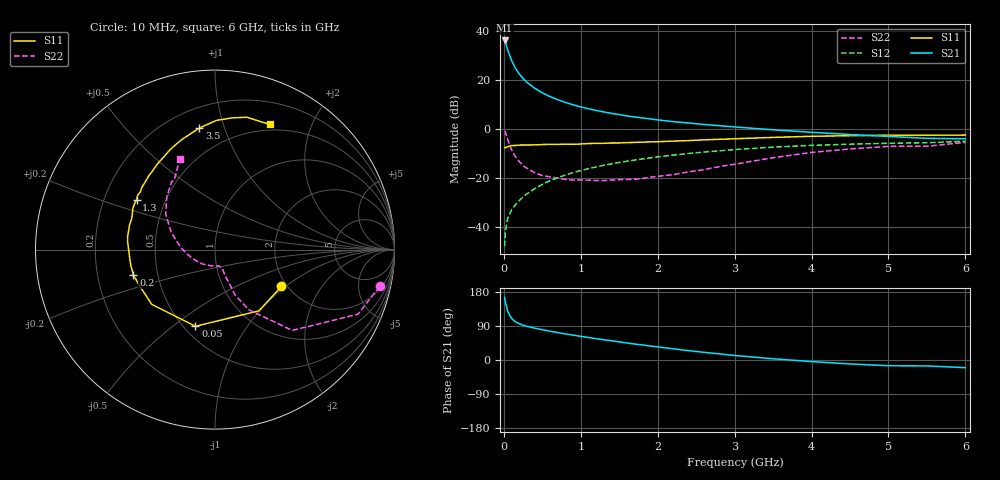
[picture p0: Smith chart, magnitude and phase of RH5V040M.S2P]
! SIEMENS Small Signal Semiconductors
! BFR106
! Si NPN RF Bipolar Junction Transistor in SOT23
! VCE = 5 V  IC = 40 mA
! Common Emitter S-Parameters:  August  1996
# GHz  S  MA  R  50
!  f  S11  S21  S12  S22
! GHz  MAG  ANG  MAG  ANG  MAG  ANG  MAG  ANG
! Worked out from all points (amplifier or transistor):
!   36 points, 10 MHz to 6 GHz, reference 50 ohm
!   highest |S21| = 36.3 dB at 10 MHz (marker M1)
!   |S21| within 3 dB of that: start of sweep to 41.81 MHz
!   unconditionally stable (mu >= 1): 274.4 MHz to 2.238 GHz
!   at 250 MHz: K = 0.98, MSG = 24.2 dB, |S12| = -27.7 dB
!   at 1.4 GHz: K = 1.05, MAG = 8.9 dB, |S12| = -14.1 dB
!   at 6 GHz: K = 0.98, MSG = 0.5 dB, |S12| = -4.9 dB
!   S11 on the Smith chart (normalised r, x): 10 MHz: 1.87, -0.93; 50 MHz: 0.57, -0.61; 200 MHz: 0.36, -0.13; 1.3 GHz: 0.34, +0.26; 3.5 GHz: 0.33, +0.83; 6 GHz: 0.43, +1.44
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0.01  0.4231 -29.0  65.3 164.9  0.0041 83.9  0.9397 -12.6
0.02  0.4201 -54.3  59.77 153.0  0.0081 71.0  0.8744 -24.3
0.05  0.441 -104.3  41.98 128.0  0.0154 60.7  0.6227 -46.3
0.1  0.4661 -139.1  25.43 109.9  0.0224 58.9  0.384 -60.7
0.15  0.4665 -154.7  17.68 100.8  0.0287 62.2  0.2767 -66.2
0.2  0.476 -162.6  13.56 95.7  0.035 65.2  0.2203 -66.8
0.25  0.4771 -169.0  10.9 91.7  0.0414 67.0  0.1807 -67.9
0.3  0.4775 -172.8  9.136 88.9  0.048 68.4  0.1605 -68.6
0.4  0.4808 -179.8  6.935 84.2  0.0612 70.6  0.1301 -68.8
0.5  0.4883 175.2  5.562 79.9  0.075 70.9  0.1136 -68.6
0.6  0.4926 171.1  4.667 76.0  0.0888 70.5  0.1067 -70.2
0.8  0.4959 163.9  3.542 68.8  0.1164 69.2  0.0948 -75.9
0.9  0.4946 160.3  3.167 65.6  0.1306 68.2  0.0916 -77.9
1.1  0.5116 153.5  2.636 59.4  0.1569 66.1  0.0915 -87.3
1.3  0.5174 147.5  2.261 53.4  0.184 63.5  0.0894 -95.7
1.7  0.5398 136.7  1.785 42.1  0.2353 58.2  0.0951 -118.6
2.2  0.5738 124.3  1.437 29.6  0.2973 50.9  0.1183 -146.7
2.8  0.6245 110.5  1.186 16.2  0.3638 41.9  0.1728 -177.6
3.5  0.6831 97.3  0.978 3.2  0.4324 31.5  0.2626 158.5
4.5  0.7407 82.4  0.783 -10.4  0.4962 16.6  0.3967 132.7
5.5  0.7568 70.3  0.655 -15.7  0.5322 6.8  0.4498 120.3
6  0.7628 66.2  0.641 -20.2  0.567 -0.4  0.5406 111.3
